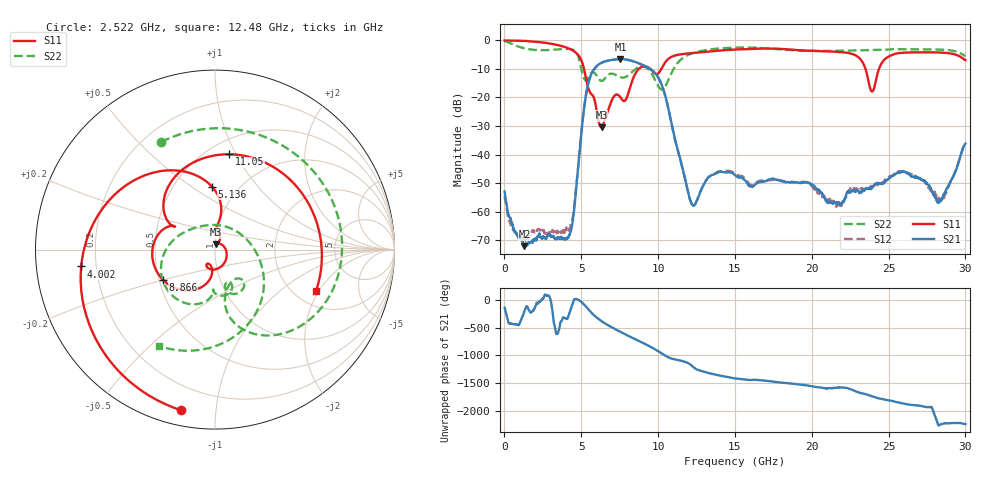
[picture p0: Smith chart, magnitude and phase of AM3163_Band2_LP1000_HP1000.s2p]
!Agilent Technologies,E8364B,MY43040894,A.07.50.67
!Agilent E8364B: A.07.50.67
!Date: Thursday, August 20, 2020 11:15:30
!Correction: S11(Full 2 Port(1,2))
!S21(Full 2 Port(1,2))
!S12(Full 2 Port(1,2))
!S22(Full 2 Port(1,2))
!S2P File: Measurements: S11, S21, S12, S22:
# Hz S  dB  R 50
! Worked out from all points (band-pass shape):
!   3201 points, 10 MHz to 30 GHz, reference 50 ohm
!   highest |S21| = -6.58 dB at 7.545 GHz (marker M1); lowest = -72.1 dB at 1.303 GHz (marker M2)
!   |S21| within 3 dB of the highest: 5.911 GHz to 9.346 GHz (3.435 GHz wide, 45 % of centre)
!   lowest |S11| = -30.5 dB at 6.317 GHz (marker M3), VSWR 1.06, Z = 50.5 + j2.95 ohm
!   |S11| at or under -10 dB: 5.178 GHz to 8.747 GHz (3.569 GHz wide, 51.3 % of centre); 9.485 GHz to 10.21 GHz (728.5 MHz wide, 7.4 % of centre); 23.5 GHz to 24.38 GHz (879.9 MHz wide, 3.68 % of centre)
!   |S22| runs from -17.3 to -0.3 dB; largest |S21 - S12| = 0.0049
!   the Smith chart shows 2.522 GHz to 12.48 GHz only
!   S11 on the Smith chart (normalised r, x): 2.522 GHz: 0.07, -0.81; 4.002 GHz: 0.14, -0.06; 5.136 GHz: 0.76, +0.61; 8.866 GHz: 0.52, -0.20; 11.05 GHz: 0.63, +0.94; 12.48 GHz: 2.56, -1.89
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1e7  -0.05 -2.8  -52.96 -139.0  -54.51 17.4  -0.27 -10.0
6.098e8  -0.08 -24.0  -66.49 -76.9  -66.03 -72.3  -1.58 -79.8
1.303319e9  -0.20 -51.7  -72.11 164.3  -69.99 115.7  -2.80 -149.7
2.521662e9  -0.77 -101.9  -68.56 20.3  -66.50 -107.0  -3.47 116.5
4.002419e9  -2.48 -172.8  -69.36 24.0  -65.99 111.0  -2.98 13.3
4.471012e9  -3.64 157.1  -62.28 -35.3  -61.09 -31.1  -3.37 -27.2
5.014581e9  -7.12 106.7  -31.82 -36.6  -31.83 -36.9  -10.38 -79.4
5.136416e9  -9.10 92.7  -25.81 -69.2  -25.82 -69.4  -12.85 -72.6
6.317272e9  -30.53 78.6  -7.83 -20.2  -7.86 -20.3  -14.22 -69.6
7.544988e9  -19.98 -118.5  -6.58 145.1  -6.61 145.0  -12.91 -92.8
8.866422e9  -9.48 -150.2  -8.34 -35.1  -8.35 -35.2  -9.18 -125.8
1.000979e10  -11.56 150.8  -13.05 154.1  -13.00 154.1  -16.04 127.2
1.105007e10  -5.40 81.4  -33.57 10.6  -33.69 8.9  -9.68 -33.8
1.248397e10  -4.32 -22.5  -56.55 -168.8  -56.45 -165.6  -4.12 -120.2
1.5005e10  -3.23 -140.6  -47.22 24.2  -46.75 25.0  -2.54 147.0
1.77697e10  -2.94 95.7  -48.87 -43.7  -49.05 -47.2  -3.09 41.4
2.000958e10  -3.71 -19.0  -50.55 -117.7  -51.09 -122.1  -3.70 -41.0
2.28024e10  -5.12 -138.9  -52.98 157.7  -52.00 157.7  -3.56 -122.0
2.392702e10  -17.92 -140.4  -51.55 62.5  -50.68 62.1  -3.39 -150.2
2.500479e10  -5.67 -136.4  -48.57 -9.6  -47.92 -11.5  -3.23 -176.0
2.830369e10  -4.26 110.3  -56.78 -96.7  -55.41 32.6  -3.23 98.5
3e10  -6.93 47.2  -36.22 -81.3  -35.89 -80.2  -5.51 47.7
